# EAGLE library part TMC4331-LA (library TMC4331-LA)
Motion Controller, no ENC; QFN32(4x4)
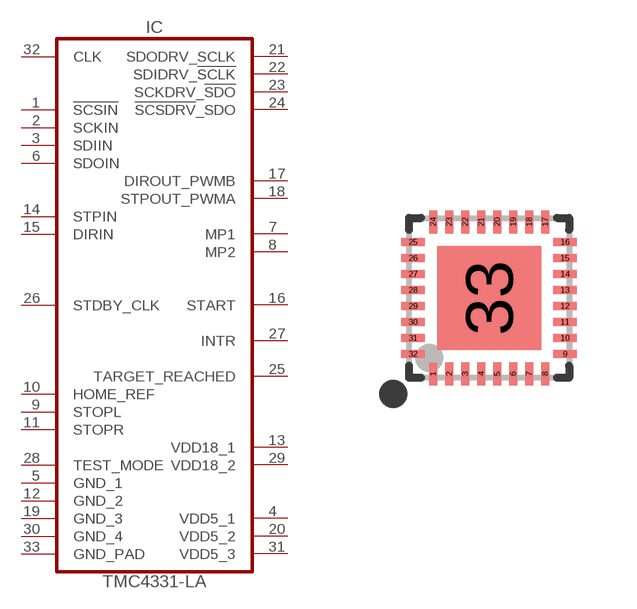
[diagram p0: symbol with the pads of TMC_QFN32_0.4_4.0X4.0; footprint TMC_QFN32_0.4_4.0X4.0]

Designator prefix IC

## TMC4331-LA (DESCRIPTION: Motion Controller, no ENC; QFN32(4x4); GEOMETRY_HEIGHT: 0_9mm; MANUFACTURER: TRINAMIC; ORDERCODE-MANU1: TMC4331-LA; VALUE: TMC4331-LA)  [TMC_QFN32_0.4_4.0X4.0]
1  !SCSIN  in
2  SCKIN  in
3  SDIIN  in
4  VDD5_1  pwr
5  GND_1  pwr
6  SDOIN  out
7  MP1  in
8  MP2
9  STOPL  in
10  HOME_REF  in
11  STOPR  in
12  GND_2  pwr
13  VDD18_1  pwr
14  STPIN  in
15  DIRIN  in
16  START
17  DIROUT_PWMB  out
18  STPOUT_PWMA  out
19  GND_3  pwr
20  VDD5_2  pwr
21  SDODRV_SCLK
22  SDIDRV_!SCLK  in
23  SCKDRV_!SDO  out
24  !SCSDRV!_SDO  out
25  TARGET_REACHED  out
26  STDBY_CLK  out
27  INTR  out
28  TEST_MODE  in
29  VDD18_2  pwr
30  GND_4  pwr
31  VDD5_3  pwr
32  CLK  in
33  GND_PAD  pwr

## Footprint TMC_QFN32_0.4_4.0X4.0 (pad centres in mm)
smd 0.2 x 0.58: 1 -1.4,-1.9; 2 -1,-1.9; 3 -0.6,-1.9; 4 -0.2,-1.9; 5 0.2,-1.9; 6 0.6,-1.9; 7 1,-1.9; 8 1.4,-1.9; 17 1.4,1.9; 18 1,1.9; 19 0.6,1.9; 20 0.2,1.9; 21 -0.2,1.9; 22 -0.6,1.9; 23 -1,1.9; 24 -1.4,1.9
smd 0.58 x 0.2: 9 1.9,-1.4; 10 1.9,-1; 11 1.9,-0.6; 12 1.9,-0.2; 13 1.9,0.2; 14 1.9,0.6; 15 1.9,1; 16 1.9,1.4; 25 -1.9,1.4; 26 -1.9,1; 27 -1.9,0.6; 28 -1.9,0.2; 29 -1.9,-0.2; 30 -1.9,-0.6; 31 -1.9,-1; 32 -1.9,-1.4
smd 2.6 x 2.6: 33 0,0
